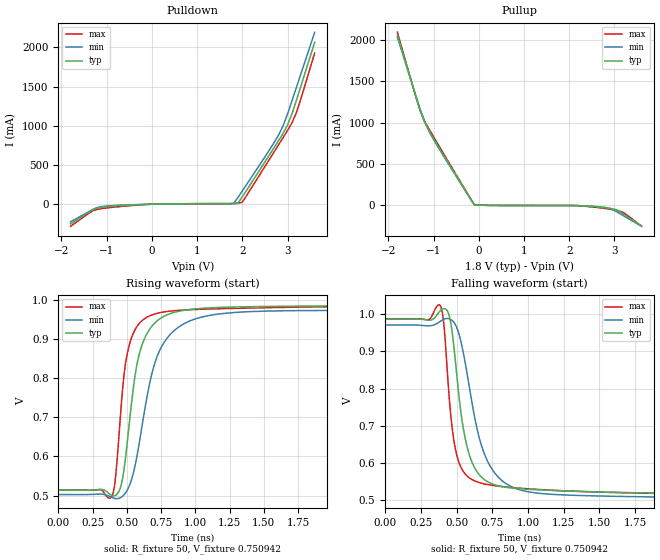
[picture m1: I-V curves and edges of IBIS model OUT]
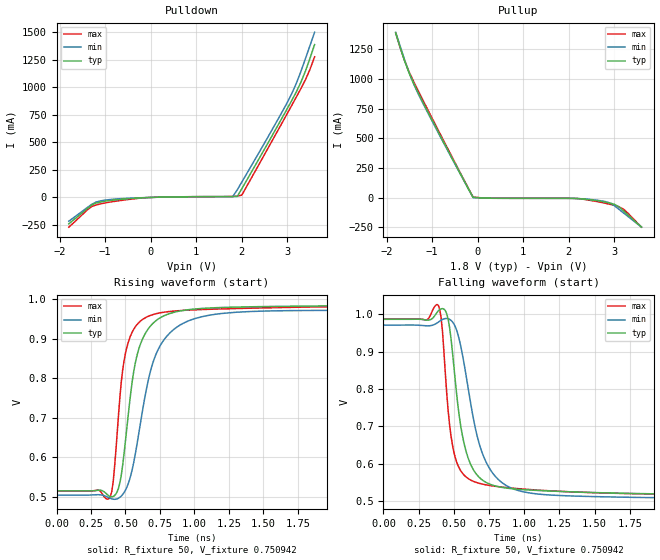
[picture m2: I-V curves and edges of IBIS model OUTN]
|   IBIS File of SG2520VGN E
|   LVDS, Vcc=1.8V, Io=4.5mA, fo<=212.5MHz
[IBIS Ver]   3.2
[File Name]   sg2520vgn_45m_18v.ibs
[File Rev]   1.0
[Date]   Sep. 17, 2020
[Source]
Fairchild Ensigna Lab's Method
[Notes]
Created by Minoru Kozaki
[Disclaimer]
Seiko Epson Corporation makes no warranty with respect to the
information contained herein.
[Copyright]
Copyright(C) 2020, Seiko Epson Corporation. All rights reserved.
|   Component
[Component]   SG2520VGN
[Manufacturer]  Seiko Epson Corporation
[Package]
R_pkg   17.7m   NA   NA
L_pkg   235p   NA   NA
C_pkg   208f   NA   NA
[Pin]   signal_name   model_name   R_pin   L_pin   C_pin
1   OE/ST   NC
2   NC   NC
3   GND   GND
4   OUT   OUT   17.7m   235p   208f
5   OUTN   OUTN   10.4m   129p   221f
6   VCC   POWER
[Diff Pin] inv_pin  vdiff  tdelay_typ
4   5   0   0
| Models and submodels in the file (2): OUT (Output), OUTN (Output)
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|   Model OUT
[Model]   OUT
Model_type   Output
Polarity   Non-Inverting
Vref = 0.75
Vmeas = 0.75
Rref = 50
Cref = 0
C_comp   4.5p   4.5p   4.5p
[Temperature Range]   25   105   -40
[Voltage Range]   1.8   1.71   1.89
[Pullup Reference]   1.8   1.71   1.89
[Pulldown Reference]   0   0   0
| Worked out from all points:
|   slope of the pulldown table from 0 to 0.27 V, typ, clamps not added: 82.4 ohm
|   slope of the pullup table from 0 to 0.27 V, typ, clamps not added: 63.8 ohm
|   falling waveform, R_fixture 50, V_fixture 0.750942: 20-80 % time 114ps typ, 170ps min, 83ps max; typ from 0.987 V to 0.514 V
|   rising waveform, R_fixture 50, V_fixture 0.750942: 20-80 % time 125ps typ, 179ps min, 91.8ps max; typ from 0.514 V to 0.986 V
[Pullup]
-1.8V     2.06A      2.034A     2.094A
-1.4V     1.329A     1.339A     1.328A
-1.3V     1.152A     1.166A     1.152A
-1.2V     1.007A     1.011A     1.022A
-1.1V     899.9mA    891.8mA    921.8mA
-1V       805.7mA    793.5mA    827.8mA
-100mV    2.963mA    1.882mA    6.416mA
2.1V      -5.449mA   -5.565mA   -5.304mA
2.8V      -31.96mA   -29.08mA   -41.84mA
3V        -49.97mA   -64.35mA   -57.97mA
3.2V      -109.2mA   -129.3mA   -90.72mA
3.6V      -256.7mA   -257.3mA   -254.5mA
[Pulldown]
-1.8V     -250.1mA   -224.3mA   -281.7mA
-1.3V     -68.95mA   -63.8mA    -81.92mA
-1.1V     -38.85mA   -29.58mA   -55.53mA
0V        -69.51uA   -61.58uA   -72.46uA
1.8V      7.367mA    7.053mA    9.466mA
1.9V      8.809mA    83.45mA    13.06mA
2V        95.48mA    169.3mA    25.88mA
2.8V      809.3mA    880.6mA    756.3mA
2.9V      902.7mA    997.2mA    847.9mA
3V        1.01A      1.15A      940.8mA
3.2V      1.332A     1.496A     1.174A
3.6V      2.064A     2.193A     1.928A
[Falling Waveform]
R_fixture = 50
V_fixture = 0.750942
V_fixture_min = 0.737533
V_fixture_max = 0.751314
0s        986.8mV    971.3mV    987.6mV
380ps     1.007V     979.6mV    1.026V
430ps     1.012V     988.8mV    874.6mV
460ps     975.3mV    986mV      723.6mV
500ps     840.6mV    965.4mV    622.1mV
570ps     648.2mV    847.5mV    565.6mV
660ps     567.2mV    664.8mV    546.5mV
800ps     537.3mV    558mV      536.8mV
1.05ns    527.6mV    519mV      528.7mV
4ns       514.1mV    503.3mV    513.7mV
[Rising Waveform]
R_fixture = 50
V_fixture = 0.750942
V_fixture_min = 0.737533
V_fixture_max = 0.751314
0s        513.6mV    502.5mV    513.4mV
380ps     502mV      496.8mV    493.5mV
440ps     509mV      492.5mV    640.1mV
480ps     567.9mV    502mV      809.4mV
520ps     690mV      526.4mV    886.8mV
590ps     859.9mV    632.4mV    938.4mV
690ps     934.9mV    820.7mV    961.5mV
840ps     966.5mV    919mV      971.2mV
1.15ns    979.4mV    962.1mV    976.2mV
4ns       986.3mV    971.4mV    986.8mV
[Ramp]
R_load = 50
dV/dt_r   0.28414/125.60p   0.28052/178.51p   0.28520/92.90p
dV/dt_f   0.28414/114.00p   0.28052/169.85p   0.28520/82.85p
|   Model OUTN
[Model]   OUTN
Model_type   Output
Polarity   Inverting
Vref = 0.75
Vmeas = 0.75
Rref = 50
Cref = 0
C_comp   4.5p   4.5p   4.5p
[Temperature Range]   25   105   -40
[Voltage Range]   1.8   1.71   1.89
[Pullup Reference]   1.8   1.71   1.89
[Pulldown Reference]   0   0   0
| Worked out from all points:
|   slope of the pulldown table from 0 to 0.27 V, typ, clamps not added: 83.1 ohm
|   slope of the pullup table from 0 to 0.27 V, typ, clamps not added: 63.9 ohm
|   falling waveform, R_fixture 50, V_fixture 0.750942: 20-80 % time 115ps typ, 170ps min, 85.1ps max; typ from 0.987 V to 0.515 V
|   rising waveform, R_fixture 50, V_fixture 0.750942: 20-80 % time 125ps typ, 179ps min, 92.7ps max; typ from 0.515 V to 0.986 V
[Pullup]
-1.8V     1.387A     1.393A     1.388A
-1.6V     1.148A     1.157A     1.15A
-1.5V     1.045A     1.049A     1.056A
-1.3V     879.9mA    871.3mA    897.7mA
-800mV    507.5mA    500.1mA    520.4mA
-100mV    2.948mA    1.875mA    6.399mA
300mV     -4.231mA   -3.63mA    -4.336mA
2.1V      -5.448mA   -5.602mA   -5.302mA
2.7V      -29.1mA    -25.28mA   -38.27mA
3V        -54.58mA   -65mA      -64.48mA
3.2V      -108.9mA   -126.3mA   -94.34mA
3.6V      -246.6mA   -247.9mA   -247.2mA
[Pulldown]
-1.8V     -240mA     -216mA     -270.3mA
-1.3V     -69.93mA   -63.48mA   -83.97mA
-1V       -34.21mA   -24.57mA   -50.01mA
0V        -69.27uA   -61.42uA   -72.17uA
1.8V      7.339mA    7.026mA    9.415mA
1.9V      8.763mA    68.4mA     12.97mA
2V        78mA       138.8mA    20.8mA
2.8V      659.3mA    713.3mA    613.5mA
3.1V      882.6mA    945mA      838.2mA
3.3V      1.047A     1.146A     989.8mA
3.5V      1.266A     1.382A     1.165A
3.6V      1.389A     1.501A     1.278A
[Falling Waveform]
R_fixture = 50
V_fixture = 0.750942
V_fixture_min = 0.737533
V_fixture_max = 0.751314
0s        986.6mV    971.1mV    987.4mV
390ps     1.009V     979mV      1.024V
440ps     1.01V      988.7mV    841mV
470ps     964.8mV    986.5mV    704.6mV
510ps     823.9mV    967.4mV    616.9mV
570ps     659mV      874.1mV    570.7mV
670ps     567.7mV    667.9mV    548.6mV
800ps     539.9mV    563.9mV    539.3mV
1.05ns    529.3mV    521mV      530.5mV
4ns       515.1mV    504.6mV    514.9mV
[Rising Waveform]
R_fixture = 50
V_fixture = 0.750942
V_fixture_min = 0.737533
V_fixture_max = 0.751314
0s        514.6mV    503.8mV    514.6mV
380ps     501.8mV    497.4mV    494.8mV
430ps     506.4mV    493.5mV    615.2mV
470ps     555.8mV    501.6mV    792mV
510ps     674.6mV    524.1mV    878.4mV
580ps     852.7mV    625.5mV    934.2mV
690ps     935.6mV    829.1mV    960mV
840ps     965.7mV    920.5mV    969.6mV
1.15ns    978.4mV    961.8mV    974.9mV
4ns       986.1mV    971.3mV    986.6mV
[Ramp]
R_load = 50
dV/dt_r   0.28279/125.41p   0.27918/177.43p   0.28384/93.42p
dV/dt_f   0.28279/115.11p   0.27918/169.47p   0.28384/84.94p
